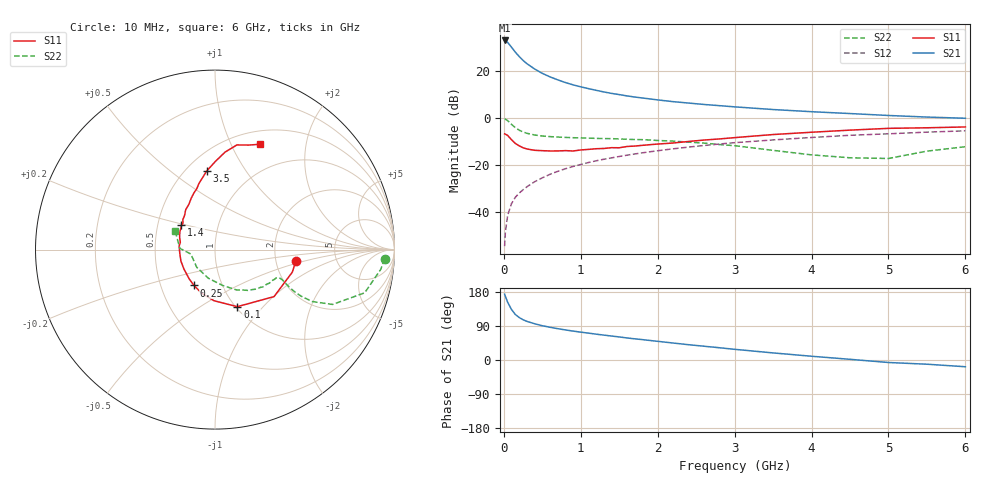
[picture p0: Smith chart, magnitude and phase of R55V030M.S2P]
! SIEMENS Small Signal Semiconductors
! BFR183
! Si NPN RF Bipolar Junction Transistor in SOT23
! VCE = 5 V  IC = 30 mA
! Common Emitter S-Parameters:  May  1996
# GHz  S  MA  R  50
!  f  S11  S21  S12  S22
! GHz  MAG  ANG  MAG  ANG  MAG  ANG  MAG  ANG
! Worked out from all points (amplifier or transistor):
!   36 points, 10 MHz to 6 GHz, reference 50 ohm
!   highest |S21| = 32.7 dB at 10 MHz (marker M1)
!   |S21| within 3 dB of that: start of sweep to 103 MHz
!   unconditionally stable (mu >= 1): 467.4 MHz to 2.383 GHz
!   at 250 MHz: K = 0.88, MSG = 27.4 dB, |S12| = -30.5 dB
!   at 1.4 GHz: K = 1.04, MAG = 12.4 dB, |S12| = -17.0 dB
!   at 6 GHz: K = 0.90, MSG = 2.7 dB, |S12| = -5.5 dB
!   S11 on the Smith chart (normalised r, x): 10 MHz: 2.59, -0.42; 100 MHz: 1.02, -0.73; 250 MHz: 0.74, -0.31; 1.4 GHz: 0.66, +0.19; 3.5 GHz: 0.63, +0.68; 6 GHz: 0.65, +1.29
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0.01  0.4542 -8.1  43.36 173.7  0.0019 90.4  0.9458 -3.1
0.02  0.4489 -16.2  42.84 167.8  0.0038 80.8  0.9302 -6.8
0.05  0.4205 -38.5  39.38 152.3  0.0086 78.1  0.868 -16.1
0.1  0.3415 -68.6  31.15 133.1  0.0152 71.6  0.723 -25.0
0.15  0.2848 -91.2  24.45 120.0  0.0207 70.0  0.6142 -28.1
0.2  0.2535 -107.4  19.76 112.0  0.0253 70.6  0.5439 -28.4
0.25  0.2313 -120.4  16.39 106.2  0.0298 71.2  0.4982 -27.8
0.3  0.2177 -131.2  13.97 101.9  0.0345 72.2  0.4679 -27.0
0.4  0.2042 -147.7  10.79 95.7  0.044 73.6  0.4308 -25.2
0.5  0.2004 -161.1  8.71 90.4  0.0533 73.7  0.4098 -24.2
0.6  0.1975 -169.2  7.343 86.4  0.0633 73.6  0.3979 -23.8
0.7  0.1978 -178.2  6.347 82.7  0.0731 73.4  0.39 -23.9
0.8  0.2009 174.5  5.565 79.4  0.083 72.6  0.383 -24.2
0.9  0.1974 168.3  4.972 76.3  0.0927 72.1  0.3772 -24.6
1.1  0.2133 157.4  4.137 70.9  0.1124 70.7  0.3696 -26.8
1.4  0.232 143.9  3.279 63.2  0.141 68.0  0.3602 -30.2
1.7  0.2509 133.5  2.747 55.9  0.1705 64.8  0.3452 -34.4
2.2  0.2914 119.9  2.191 44.8  0.2194 59.1  0.3199 -43.4
3.5  0.4405 96.0  1.491 18.7  0.3386 42.3  0.2036 -78.3
4.5  0.546 84.1  1.226 1.8  0.4247 29.7  0.1417 -135.7
5.5  0.6124 72.0  1.033 -11.1  0.4951 18.1  0.196 178.0
6  0.6374 67.0  0.974 -17.8  0.5279 10.6  0.2433 155.4
